(* Logix 5000 Rung export; software revision 33.00 *)

TYPE Banner_IOL_Device :
STRUCT
   Initial_Global_Read : BOOL;
   Command : SINT;
   Data : Banner_IOL_Device_Index;
   Reset : BOOL;
END_STRUCT
END_TYPE

TYPE Banner_IOL_Device_Index :
STRUCT
   Index : Banner_IOL_Device_SubIndex[32];
END_STRUCT
END_TYPE

TYPE Banner_IOL_Device_SubIndex :
STRUCT
   Sub : DINT[34];
END_STRUCT
END_TYPE

TYPE Banner_IOL_Rules :
STRUCT
   Byte_Pos : SINT;   // Byte Position to read from or write data to.
   Multi : SINT;   // Determines if a multiple byte length index is being accessed. Use 2 for 2 bytes length, 3 for 3 byte length, etc..
   Sub_Index : SINT;
   Signed : SINT;   // 0=Unsigned, 1=Signed
END_STRUCT
END_TYPE

TYPE Banner_IOL_Rules_Array :
STRUCT
   Length : DINT;
   Settings : Banner_IOL_Rules_SettingsArray[32];
END_STRUCT
END_TYPE

TYPE Banner_IOL_Rules_SettingsArray :
STRUCT
   Index : DINT;
   Num_Op : INT;   // Number of Operations to read/write Index.
   Total_Bytes : INT;
   RW : SINT;   // 0 = Read Only, 1 = Write Only, 2 = Read or Write
   Rules : Banner_IOL_Rules[34];   // Sub Index Position in IODD.
END_STRUCT
END_TYPE

VAR_GLOBAL   (* controller tags *)
   S100_IOLM1_01 : Banner_IOL_Device;
        .DATA.INDEX[2]   // Direct Parameters 1 (ro)
        .DATA.INDEX[2].SUB[1]   // Reserved
        .DATA.INDEX[2].SUB[2]   // Master Cycle Time
        .DATA.INDEX[2].SUB[3]   // Min Cycle Time
        .DATA.INDEX[2].SUB[4]   // M Sequence Capability
        .DATA.INDEX[2].SUB[5]   // IO-Link Verson ID
        .DATA.INDEX[2].SUB[6]   // Process Data Input Length
        .DATA.INDEX[2].SUB[7]   // Process Data Output Length
        .DATA.INDEX[2].SUB[8]   // Vendor ID
        .DATA.INDEX[2].SUB[9]   // Device ID
        .DATA.INDEX[3]   // Standard Command (wo)
        .DATA.INDEX[3].SUB[1]   // Standard Command
        .DATA.INDEX[4]   // Device Locks
        .DATA.INDEX[4].SUB[1]   // Parameter Access Lock / Data Storage Lock / Local Parameterization Lock / Local User Interface Lock
        .DATA.INDEX[5]   // Serial Number (ro)
        .DATA.INDEX[5].SUB[1]   // SN1
        .DATA.INDEX[5].SUB[2]   // SN2
        .DATA.INDEX[5].SUB[3]   // SN3
        .DATA.INDEX[5].SUB[4]   // SN4
        .DATA.INDEX[5].SUB[5]   // SN5
        .DATA.INDEX[5].SUB[6]   // SN6
        .DATA.INDEX[5].SUB[7]   // SN7
        .DATA.INDEX[5].SUB[8]   // SN8
        .DATA.INDEX[5].SUB[9]   // SN9
        .DATA.INDEX[5].SUB[10]   // SN10
        .DATA.INDEX[5].SUB[11]   // SN11
        .DATA.INDEX[5].SUB[12]   // SN12
        .DATA.INDEX[5].SUB[13]   // SN13
        .DATA.INDEX[5].SUB[14]   // SN14
        .DATA.INDEX[5].SUB[15]   // SN15
        .DATA.INDEX[5].SUB[16]   // SN16
        .DATA.INDEX[6]   // Operating Mode
        .DATA.INDEX[6].SUB[1]   // Operating Mode: 0=Run, 1=4 State Full Logic, 2=Measure, 3=Timer, 4=Counter
        .DATA.INDEX[7]   // Additional Settings
        .DATA.INDEX[7].SUB[1]   // Custom Intensity: 0 to 100%
        .DATA.INDEX[7].SUB[2]   // Custom Flash Rate: 5 to 200 (.5 to 20 Hz)
        .DATA.INDEX[7].SUB[3]   // Custom Display Intensity: 0 to 100 %
        .DATA.INDEX[7].SUB[4]   // Custom Display Scroll Speed: 0 to 255
        .DATA.INDEX[8]   // Display Settings
        .DATA.INDEX[8].SUB[1]   // Text Color / Intensity / Scroll Direction / Scroll Speed / Font Size: see iodd file for more information
        .DATA.INDEX[8].SUB[2]   // Scroll Mode Line 1 / Line 2 / Scynch Scroll / Orientation / Deadspace: see iodd file for more information
        .DATA.INDEX[8].SUB[3]   // Deadspace Value: 0 to 29. The amount of deadspace in columns to insert between the start and end of display strings
        .DATA.INDEX[8].SUB[4]   // Horizontal Justification / Vertial Justification: see iodd file for more information
        .DATA.INDEX[9]   // Timer Settings
        .DATA.INDEX[9].SUB[1]   // Value: Value to count up to or down from.
        .DATA.INDEX[9].SUB[2]   // Timer Unit Type: 0=Days, 1=Hours, 2=Minutes, 3=Seconds, 4=Deci Seconds, 5=Centi Seconds, 6=Milli Seconds
        .DATA.INDEX[9].SUB[3]   // Timer Count Type: 0=Down, 1=Up
        .DATA.INDEX[9].SUB[4]   // Reset Button: 0=Disabled, 1=Button 1, 2=Button 2, 3=Button 3. 4=Button 4, 5=Button 5
        .DATA.INDEX[9].SUB[5]   // Count Inrement Button: 0=Disabled, 1=Button 1, 2=Button 2, 3=Button 3. 4=Button 4, 5=Button 5
        .DATA.INDEX[9].SUB[6]   // Count Decrement Button: 0=Disabled, 1=Button 1, 2=Button 2, 3=Button 3. 4=Button 4, 5=Button 5
        .DATA.INDEX[9].SUB[7]   // Run/Pause Button: 0=Disabled, 1=Button 1, 2=Button 2, 3=Button 3. 4=Button 4, 5=Button 5
        .DATA.INDEX[9].SUB[8]   // Enable Auto Reload: 0=Disabled, 1=Enabled
        .DATA.INDEX[10]   // Measure General Configuration
        .DATA.INDEX[10].SUB[1]   // Filtering: 0=Off, 1=Low, 2=Medium, 3=High
        .DATA.INDEX[10].SUB[2]   // Hysteresis: 0=Off, 1=Low, 2=Medium, 3=High
        .DATA.INDEX[10].SUB[3]   // MTC Mode Data Label 1: DINT representation of a ASCII String
        .DATA.INDEX[10].SUB[4]   // MTC Mode Data Label 2: DINT representation of a ASCII String
        .DATA.INDEX[10].SUB[5]   // MTC Mode Data Label 3: DINT representation of a ASCII String
        .DATA.INDEX[10].SUB[6]   // MTC Mode Data Label 4: DINT representation of a ASCII String
        .DATA.INDEX[10].SUB[7]   // Display Value: 0=Disabled, 1=Enabled
        .DATA.INDEX[10].SUB[8]   // Display Data Label: 0=Disabled, 1=Enabled
        .DATA.INDEX[10].SUB[9]   // Display Bar Graph: 0=Disabled, 1=Enabled
        .DATA.INDEX[10].SUB[10]   // Gauge Mode: 0=Disabled, 1=Enabled
        .DATA.INDEX[10].SUB[11]   // Guage Mode Direction: 0=False, 1=Enabled
        .DATA.INDEX[10].SUB[12]   // Gauge Mode Shift: 0=LED1, 1=LED2, 2=LED3, 3=LED4, 4=LED5, 5=LED6, 6=LED7, 7=LED8, 8=LED9, 9=LED10, 10=LED11, 11=LED12, 12=LED13, 13=LED14, 14=LED15, 15=LED16
        .DATA.INDEX[10].SUB[13]   // Gauge Mode Background Color: 0=Green, 1=Red, 2=Orange, 3=Amber, 4=Yellow, 5=Lime Green, 6=Spring Green, 7=Cyan, 8=Sky Blue, 9=Blue, 10=Violet, 11=Magneta, 12=Rose, 13=White, 14=Custom 1, 15=Cusotm 2
        .DATA.INDEX[10].SUB[14]   // Gauge Mode Background Intensity: 0=High, 1=Medium, 2=Low, 3=Off, 4=Custom
        .DATA.INDEX[10].SUB[15]   // Output Scale Value Low: The lowest number to be displayed
        .DATA.INDEX[10].SUB[16]   // Output Scale Value High: The highest number to be displayed
        .DATA.INDEX[10].SUB[17]   // Input Scale Value Low: The lowest number being input by level mode process data. Set to 0 in timer/counter mode
        .DATA.INDEX[10].SUB[18]   // Input Scale Value High: The highest number being input by level mode porcess data. Set to 65535 in timer/counter mode
        .DATA.INDEX[10].SUB[19]   // Value Label: 4 characters: DINT representation of a ASCII String
        .DATA.INDEX[10].SUB[20]   // Swap Data Label and Value: 0=Disabled, 1=Enabled
        .DATA.INDEX[10].SUB[21]   // MTC Mode Display Orientation: 0=0, 1=180
        .DATA.INDEX[10].SUB[22]   // Bar Graph Height: 1 to 16=Bar Graph Packages
        .DATA.INDEX[10].SUB[23]   // MTC Mode Decimal Places: 0 to 3=Decimal Places
        .DATA.INDEX[10].SUB[24]   // MTC Mode Display as Time: 0=Disabled, 1=Enabled
        .DATA.INDEX[11]   // Measure Base Configuration
        .DATA.INDEX[11].SUB[1]   // Display Override: 0=Disabled, 1=Enabled
        .DATA.INDEX[11].SUB[2]   // Override String Line 1 - 1: Characters 1 to 4. DINT Representation of an ASCII String.
        .DATA.INDEX[11].SUB[3]   // Override String Line 1 - 2: Characters 5 to 8. DINT Representation of an ASCII String.
        .DATA.INDEX[11].SUB[4]   // Override String Line 1 - 3: Characters 9 to 12. DINT Representation of an ASCII String.
        .DATA.INDEX[11].SUB[5]   // Override String Line 1 - 4: Charcter 13. DINT Representation of an ASCII String.
        .DATA.INDEX[11].SUB[6]   // Override String Line 2 - 1: Characters 1 to 4. DINT Representation of an ASCII String.
        .DATA.INDEX[11].SUB[7]   // Override String Line 2 - 2: Characters 5 to 8. DINT Representation of an ASCII String.
        .DATA.INDEX[11].SUB[8]   // Override String Line 2 - 3: Characters 9 to 12. DINT Representation of an ASCII String.
        .DATA.INDEX[11].SUB[9]   // Override String Line 2 - 4: Charcter 13. DINT Representation of an ASCII String.
        .DATA.INDEX[11].SUB[10]   // Animation / Speed / Pulse Pattern: see iodd file for more information
        .DATA.INDEX[11].SUB[11]   // Static Sequence Value: 0 to 255
        .DATA.INDEX[11].SUB[12]   // Sequence Start Location / Top Chevron / Right Chevron / Bottom Chevron / Left Chevron: see iodd file for more information
        .DATA.INDEX[11].SUB[13]   // Color 1 / Color 1 Intensity: see iodd file for more information
        .DATA.INDEX[11].SUB[14]   // Color 2 / Color 2 Intensity: see iodd file for more information
        .DATA.INDEX[11].SUB[15]   // Direction / Haptic Feedback / Audible Type: see iodd file for more information
        .DATA.INDEX[12]   // Measure Threshold 1 Configuration
        .DATA.INDEX[12].SUB[1]   // Threshold Enable: 0=Disabled, 1=Enabled
        .DATA.INDEX[12].SUB[2]   // Threshold Value: 0 to 100 %
        .DATA.INDEX[12].SUB[3]   // Threshold Comparison: 0=Less Than, 1=Greater Than
        .DATA.INDEX[12].SUB[4]   // Threshold Override: 0=Disabled , 1=Enabled
        .DATA.INDEX[12].SUB[5]   // Display Override: 0=Disabled, 1=Enabled
        .DATA.INDEX[12].SUB[6]   // Override String Line 1-1: Characters 1 to 4. DINT representation of an ASCII String.
        .DATA.INDEX[12].SUB[7]   // Override String Line 1-2: Characters 5 to 8. DINT representation of an ASCII String.
        .DATA.INDEX[12].SUB[8]   // Override String Line 1-3: Characters 9 to 12. DINT representation of an ASCII String.
        .DATA.INDEX[12].SUB[9]   // Override String Line 1-4: Character 13. DINT representation of an ASCII String.
        .DATA.INDEX[12].SUB[10]   // Override String Line 2-1: Characters 1 to 4. DINT representation of an ASCII String.
        .DATA.INDEX[12].SUB[11]   // Override String Line 2-2: Characters 5 to 8. DINT representation of an ASCII String.
        .DATA.INDEX[12].SUB[12]   // Override String Line 2-3: Characters 9 to 12. DINT representation of an ASCII String.
        .DATA.INDEX[12].SUB[13]   // Override String Line 2-4: Character 13. DINT representation of an ASCII String.
        .DATA.INDEX[12].SUB[14]   // Animation / Speed / Pulse Pattern: see iodd file for more information
        .DATA.INDEX[12].SUB[15]   // Static Sequence Value: 0 to 255
        .DATA.INDEX[12].SUB[16]   // Sequence Start Location / Top Chevron / Right Chevron / Bottom Chevron / Left Chevron: see iodd file for more information
        .DATA.INDEX[12].SUB[17]   // Color 1 / Color 1 Intensity: see iodd file for more information
        .DATA.INDEX[12].SUB[18]   // Color 2 / Color 2 Intensity: see iodd file for more information
        .DATA.INDEX[12].SUB[19]   // Direction / Haptic Feedback / Audible Type: see iodd fiel for more information
        .DATA.INDEX[13]   // Measure Threshold 2 Configuration
        .DATA.INDEX[13].SUB[1]   // Threshold Enable: 0=Disabled, 1=Enabled
        .DATA.INDEX[13].SUB[2]   // Threshold Value: 0 to 100 %
        .DATA.INDEX[13].SUB[3]   // Threshold Comparison: 0=Less Than, 1=Greater Than
        .DATA.INDEX[13].SUB[4]   // Threshold Override: 0=Disabled , 1=Enabled
        .DATA.INDEX[13].SUB[5]   // Display Override: 0=Disabled, 1=Enabled
        .DATA.INDEX[13].SUB[6]   // Override String Line 1-1: Characters 1 to 4. DINT representation of an ASCII String.
        .DATA.INDEX[13].SUB[7]   // Override String Line 1-2: Characters 5 to 8. DINT representation of an ASCII String.
        .DATA.INDEX[13].SUB[8]   // Override String Line 1-3: Characters 9 to 12 DINT representation of an ASCII String.
        .DATA.INDEX[13].SUB[9]   // Override String Line 1-4: Character 13. DINT representation of an ASCII String.
        .DATA.INDEX[13].SUB[10]   // Override String Line 2-1: Characters 1 to 4. DINT representation of an ASCII String.
        .DATA.INDEX[13].SUB[11]   // Override String Line 2-2: Characters 5 to 8. DINT representation of an ASCII String.
        .DATA.INDEX[13].SUB[12]   // Override String Line 2-3: Characters 9 to 12. DINT representation of an ASCII String.
        .DATA.INDEX[13].SUB[13]   // Override String Line 2-4: Character 13. DINT representation of an ASCII String.
        .DATA.INDEX[13].SUB[14]   // Animation / Speed / Pulse Pattern: see iodd file for more information
        .DATA.INDEX[13].SUB[15]   // Static Sequence Value: 0 to 255
        .DATA.INDEX[13].SUB[16]   // Sequence Start Location / Top Chevron / Right Chevron / Bottom Chevron / Left Chevron: see iodd file for more information
        .DATA.INDEX[13].SUB[17]   // Color 1 / Color 1 Intensity: see iodd file for more information
        .DATA.INDEX[13].SUB[18]   // Color 2 / Color 2 Intensity: see iodd file for more information
        .DATA.INDEX[13].SUB[19]   // Direction / Haptic Feedback / Audible Type: see iodd fiel for more information
        .DATA.INDEX[14]   // Measure Threshold 3 Configuration
        .DATA.INDEX[14].SUB[1]   // Threshold Enable: 0=Disabled, 1=Enabled
        .DATA.INDEX[14].SUB[2]   // Threshold Value: 0 to 100 %
        .DATA.INDEX[14].SUB[3]   // Threshold Comparison: 0=Less Than, 1=Greater Than
        .DATA.INDEX[14].SUB[4]   // Threshold Override: 0=Disabled , 1=Enabled
        .DATA.INDEX[14].SUB[5]   // Display Override: 0=Disabled, 1=Enabled
        .DATA.INDEX[14].SUB[6]   // Override String Line 1-1: Characters 1 to 4. DINT representation of an ASCII String.
        .DATA.INDEX[14].SUB[7]   // Override String Line 1-2: Characters 5 to 8. DINT representation of an ASCII String.
        .DATA.INDEX[14].SUB[8]   // Override String Line 1-3: Characters 9 to 12. DINT representation of an ASCII String.
        .DATA.INDEX[14].SUB[9]   // Override String Line 1-4: Character 13. DINT representation of an ASCII String.
        .DATA.INDEX[14].SUB[10]   // Override String Line 2-1: Characters 1 to 4. DINT representation of an ASCII String.
        .DATA.INDEX[14].SUB[11]   // Override String Line 2-2: Characters 5 to 8. DINT representation of an ASCII String.
        .DATA.INDEX[14].SUB[12]   // Override String Line 2-3: Characters 9 to 12. DINT representation of an ASCII String.
        .DATA.INDEX[14].SUB[13]   // Override String Line 2-4: Character 13. DINT representation of an ASCII String.
        .DATA.INDEX[14].SUB[14]   // Animation / Speed / Pulse Pattern: see iodd file for more information
        .DATA.INDEX[14].SUB[15]   // Static Sequence Value: 0 to 255
        .DATA.INDEX[14].SUB[16]   // Sequence Start Location / Top Chevron / Right Chevron / Bottom Chevron / Left Chevron: see iodd file for more information
        .DATA.INDEX[14].SUB[17]   // Color 1 / Color 1 Intensity: see iodd file for more information
        .DATA.INDEX[14].SUB[18]   // Color 2 / Color 2 Intensity: see iodd file for more information
        .DATA.INDEX[14].SUB[19]   // Direction / Haptic Feedback / Audible Type: see iodd fiel for more information
        .DATA.INDEX[15]   // Measure Threshold 4 Configuration
        .DATA.INDEX[15].SUB[1]   // Threshold Enable: 0=Disabled, 1=Enabled
        .DATA.INDEX[15].SUB[2]   // Threshold Value: 0 to 100 %
        .DATA.INDEX[15].SUB[3]   // Threshold Comparison: 0=Less Than, 1=Greater Than
        .DATA.INDEX[15].SUB[4]   // Threshold Override: 0=Disabled , 1=Enabled
        .DATA.INDEX[15].SUB[5]   // Display Override: 0=Disabled, 1=Enabled
        .DATA.INDEX[15].SUB[6]   // Override String Line 1-1: Characters 1 to 4. DINT representation of an ASCII String.
        .DATA.INDEX[15].SUB[7]   // Override String Line 1-2: Characters 5 to 8. DINT representation of an ASCII String.
        .DATA.INDEX[15].SUB[8]   // Override String Line 1-3: Characters 9 to 12. DINT representation of an ASCII String.
        .DATA.INDEX[15].SUB[9]   // Override String Line 1-4: Character 13. DINT representation of an ASCII String.
        .DATA.INDEX[15].SUB[10]   // Override String Line 2-1: Characters 1 to 4. DINT representation of an ASCII String.
        .DATA.INDEX[15].SUB[11]   // Override String Line 2-2: Characters 5 to 8. DINT representation of an ASCII String.
        .DATA.INDEX[15].SUB[12]   // Override String Line 2-3: Characters 9 to 12. DINT representation of an ASCII String.
        .DATA.INDEX[15].SUB[13]   // Override String Line 2-4: Character 13. DINT representation of an ASCII String.
        .DATA.INDEX[15].SUB[14]   // Animation / Speed / Pulse Pattern: see iodd file for more information
        .DATA.INDEX[15].SUB[15]   // Static Sequence Value: 0 to 255
        .DATA.INDEX[15].SUB[16]   // Sequence Start Location / Top Chevron / Right Chevron / Bottom Chevron / Left Chevron: see iodd file for more information
        .DATA.INDEX[15].SUB[17]   // Color 1 / Color 1 Intensity: see iodd file for more information
        .DATA.INDEX[15].SUB[18]   // Color 2 / Color 2 Intensity: see iodd file for more information
        .DATA.INDEX[15].SUB[19]   // Direction / Haptic Feedback / Audible Type: see iodd fiel for more information
        .DATA.INDEX[16]   // State Parameters 1
        .DATA.INDEX[16].SUB[1]   // Animation / Speed / Pulse Pattern
        .DATA.INDEX[16].SUB[2]   // Static Sequence
        .DATA.INDEX[16].SUB[3]   // Sequence Start Location / Top Chevron / Right Chevron / Bottom Chevron / Left Chevron
        .DATA.INDEX[16].SUB[4]   // Color 1 / Color 1 Intensity
        .DATA.INDEX[16].SUB[5]   // Color 2 / Color 2 Intensity
        .DATA.INDEX[16].SUB[6]   // Direction / Haptic Feedback / Audible Type
        .DATA.INDEX[16].SUB[7]   // Line 1 Text 1: Characters 1 to 4. DINT representation of an ASCII String.
        .DATA.INDEX[16].SUB[8]   // Line 1 Text 2: Characters 5 to 8. DINT representation of an ASCII String.
        .DATA.INDEX[16].SUB[9]   // Line 1 Text 3: Characters 9 to 12. DINT representation of an ASCII String.
        .DATA.INDEX[16].SUB[10]   // Line 1 Text 4: Character 13. DINT representation of an ASCII String.
        .DATA.INDEX[16].SUB[11]   // Line 2 Text 1: Characters 1 to 4. DINT representation of an ASCII String.
        .DATA.INDEX[16].SUB[12]   // Line 2 Text 2: Characters 5 to 8. DINT representation of an ASCII String.
        .DATA.INDEX[16].SUB[13]   // Line 2 Text 3: Characters 9 to 12. DINT representation of an ASCII String.
        .DATA.INDEX[16].SUB[14]   // Line 2 Text 4: Character 13. DINT representation of an ASCII String.
        .DATA.INDEX[17]   // State Parameters 2
        .DATA.INDEX[17].SUB[1]   // Animation / Speed / Pulse Pattern
        .DATA.INDEX[17].SUB[2]   // Static Sequence
        .DATA.INDEX[17].SUB[3]   // Sequence Start Location / Top Chevron / Right Chevron / Bottom Chevron / Left Chevron
        .DATA.INDEX[17].SUB[4]   // Color 1 / Color 1 Intensity
        .DATA.INDEX[17].SUB[5]   // Color 2 / Color 2 Intensity
        .DATA.INDEX[17].SUB[6]   // Direction / Haptic Feedback / Audible Type
        .DATA.INDEX[17].SUB[7]   // Line 1 Text 1: Characters 1 to 4. DINT representation of an ASCII String.
        .DATA.INDEX[17].SUB[8]   // Line 1 Text 2: Characters 5 to 8. DINT representation of an ASCII String.
        .DATA.INDEX[17].SUB[9]   // Line 1 Text 3: Characters 9 to 12. DINT representation of an ASCII String.
        .DATA.INDEX[17].SUB[10]   // Line 1 Text 4: Character 13. DINT representation of an ASCII String.
        .DATA.INDEX[17].SUB[11]   // Line 2 Text 1: Characters 1 to 4. DINT representation of an ASCII String.
        .DATA.INDEX[17].SUB[12]   // Line 2 Text 2: Characters 5 to 8. DINT representation of an ASCII String.
        .DATA.INDEX[17].SUB[13]   // Line 2 Text 3: Characters 9 to 12. DINT representation of an ASCII String.
        .DATA.INDEX[17].SUB[14]   // Line 2 Text 4: Character 13. DINT representation of an ASCII String.
        .DATA.INDEX[18]   // State Parameters 3
        .DATA.INDEX[18].SUB[1]   // Animation / Speed / Pulse Pattern
        .DATA.INDEX[18].SUB[2]   // Static Sequence
        .DATA.INDEX[18].SUB[3]   // Sequence Start Location / Top Chevron / Right Chevron / Bottom Chevron / Left Chevron
        .DATA.INDEX[18].SUB[4]   // Color 1 / Color 1 Intensity
        .DATA.INDEX[18].SUB[5]   // Color 2 / Color 2 Intensity
        .DATA.INDEX[18].SUB[6]   // Direction / Haptic Feedback / Audible Type
        .DATA.INDEX[18].SUB[7]   // Line 1 Text 1: Characters 1 to 4. DINT representation of an ASCII String.
        .DATA.INDEX[18].SUB[8]   // Line 1 Text 2: Characters 5 to 8. DINT representation of an ASCII String.
        .DATA.INDEX[18].SUB[9]   // Line 1 Text 3: Characters 9 to 12. DINT representation of an ASCII String.
        .DATA.INDEX[18].SUB[10]   // Line 1 Text 4: Character 13. DINT representation of an ASCII String.
        .DATA.INDEX[18].SUB[11]   // Line 2 Text 1: Characters 1 to 4. DINT representation of an ASCII String.
        .DATA.INDEX[18].SUB[12]   // Line 2 Text 2: Characters 5 to 8. DINT representation of an ASCII String.
        .DATA.INDEX[18].SUB[13]   // Line 2 Text 3: Characters 9 to 12. DINT representation of an ASCII String.
        .DATA.INDEX[18].SUB[14]   // Line 2 Text 4: Character 13. DINT representation of an ASCII String.
        .DATA.INDEX[19]   // State Parameters 4
        .DATA.INDEX[19].SUB[1]   // Animation / Speed / Pulse Pattern
        .DATA.INDEX[19].SUB[2]   // Static Sequence
        .DATA.INDEX[19].SUB[3]   // Sequence Start Location / Top Chevron / Right Chevron / Bottom Chevron / Left Chevron
        .DATA.INDEX[19].SUB[4]   // Color 1 / Color 1 Intensity
        .DATA.INDEX[19].SUB[5]   // Color 2 / Color 2 Intensity
        .DATA.INDEX[19].SUB[6]   // Direction / Haptic Feedback / Audible Type
        .DATA.INDEX[19].SUB[7]   // Line 1 Text 1: Characters 1 to 4. DINT representation of an ASCII String.
        .DATA.INDEX[19].SUB[8]   // Line 1 Text 2: Characters 5 to 8. DINT representation of an ASCII String.
        .DATA.INDEX[19].SUB[9]   // Line 1 Text 3: Characters 9 to 12. DINT representation of an ASCII String.
        .DATA.INDEX[19].SUB[10]   // Line 1 Text 4: Character 13. DINT representation of an ASCII String.
        .DATA.INDEX[19].SUB[11]   // Line 2 Text 1: Characters 1 to 4. DINT representation of an ASCII String.
        .DATA.INDEX[19].SUB[12]   // Line 2 Text 2: Characters 5 to 8. DINT representation of an ASCII String.
        .DATA.INDEX[19].SUB[13]   // Line 2 Text 3: Characters 9 to 12. DINT representation of an ASCII String.
        .DATA.INDEX[19].SUB[14]   // Line 2 Text 4: Character 13. DINT representation of an ASCII String.
        .DATA.INDEX[20]   // Custom Color 1
        .DATA.INDEX[20].SUB[1]   // Red: 0 to 255
        .DATA.INDEX[20].SUB[2]   // Green: 0 to 255
        .DATA.INDEX[20].SUB[3]   // Blue: 0 to 255
        .DATA.INDEX[21]   // Custom Color 2
        .DATA.INDEX[21].SUB[1]   // Red: 0 to 255
        .DATA.INDEX[21].SUB[2]   // Green: 0 to 255
        .DATA.INDEX[21].SUB[3]   // Blue: 0 to 255
        .DATA.INDEX[22]   // User Input Settings
        .DATA.INDEX[22].SUB[1]   // Touch Sensitivity / Only First Config: see iodd file for more information
        .DATA.INDEX[22].SUB[2]   // Button 1 Function / Mute Enable / Group Override: see iodd file for more information
        .DATA.INDEX[22].SUB[3]   // Button 1 On Delay
        .DATA.INDEX[22].SUB[4]   // Button 2 Function / Mute Enable / Group Override: see iodd file for more information
        .DATA.INDEX[22].SUB[5]   // Button 2 On Delay
        .DATA.INDEX[22].SUB[6]   // Button 3 Function / Mute Enable / Group Override: see iodd file for more information
        .DATA.INDEX[22].SUB[7]   // Button 3 On Delay
        .DATA.INDEX[22].SUB[8]   // Button 4 Function / Mute Enable / Group Override: see iodd file for more information
        .DATA.INDEX[22].SUB[9]   // Button 4 On Delay
        .DATA.INDEX[22].SUB[10]   // Button 5 Function / Mute Enable / Group Override: see iodd file for more information
        .DATA.INDEX[22].SUB[11]   // Button 5 On Delay
        .DATA.INDEX[23]   // Output Settings
        .DATA.INDEX[23].SUB[1]   // Output State: 0=Normally Closed, 1=Normally Open
        .DATA.INDEX[23].SUB[2]   // Button 1 Off Delay Type / Audible Override / Haptic Override: see iodd file for more information
        .DATA.INDEX[23].SUB[3]   // Button 1 Off Delay
        .DATA.INDEX[23].SUB[4]   // Button 2 Off Delay Type / Audible Override / Haptic Override: see iodd file for more information
        .DATA.INDEX[23].SUB[5]   // Button 2 Off Delay
        .DATA.INDEX[23].SUB[6]   // Button 3 Off Delay Type / Audible Override / Haptic Override: see iodd file for more information
        .DATA.INDEX[23].SUB[7]   // Button 3 Off Delay
        .DATA.INDEX[23].SUB[8]   // Button 4 Off Delay Type / Audible Override / Haptic Override: see iodd file for more information
        .DATA.INDEX[23].SUB[9]   // Button 4 Off Delay
        .DATA.INDEX[23].SUB[10]   // Button 5 Off Delay Type / Audible Override / Haptic Override: see iodd file for more information
        .DATA.INDEX[23].SUB[11]   // Button 5 Off Delay
        .DATA.INDEX[24]   // Custom Audible Settings
        .DATA.INDEX[24].SUB[1]   // Custom Type / Custom Sweep Type / Custom Freq 1 / Custom Freq 2: see iodd file for more information
   S100_Rules : Banner_IOL_Rules_Array;
        .SETTINGS[2]   // Direct Parameters 1
        .SETTINGS[2].RULES[0]   // Reserved
        .SETTINGS[2].RULES[1]   // Master Cycle Time
        .SETTINGS[2].RULES[2]   // Min Cycle Time
        .SETTINGS[2].RULES[3]   // M-Sequence Capability
        .SETTINGS[2].RULES[4]   // IO-Link ID
        .SETTINGS[2].RULES[5]   // Process Data Input Length
        .SETTINGS[2].RULES[6]   // Process Data Output Length
        .SETTINGS[2].RULES[7]   // Vendor ID
        .SETTINGS[2].RULES[8]   // Device ID
        .SETTINGS[3]   // Standard Command
        .SETTINGS[3].RULES[0]   // Standard Command
        .SETTINGS[4]   // Device Access Locks
        .SETTINGS[4].RULES[0]   // Parameter Access Locks / Data Storage Lock / Local Parameterization Lock / Local User Interface Lock
        .SETTINGS[5]   // Serial Number
        .SETTINGS[5].RULES[0]   // SN1
        .SETTINGS[5].RULES[1]   // SN2
        .SETTINGS[5].RULES[2]   // SN3
        .SETTINGS[5].RULES[3]   // SN4
        .SETTINGS[5].RULES[4]   // SN5
        .SETTINGS[5].RULES[5]   // SN6
        .SETTINGS[5].RULES[6]   // SN7
        .SETTINGS[5].RULES[7]   // SN8
        .SETTINGS[5].RULES[8]   // SN9
        .SETTINGS[5].RULES[9]   // SN10
        .SETTINGS[5].RULES[10]   // SN11
        .SETTINGS[5].RULES[11]   // SN12
        .SETTINGS[5].RULES[12]   // SN13
        .SETTINGS[5].RULES[13]   // SN14
        .SETTINGS[5].RULES[14]   // SN15
        .SETTINGS[5].RULES[15]   // SN16
        .SETTINGS[6]   // Operating Mode
        .SETTINGS[6].RULES[0]   // Operating Mode
        .SETTINGS[7]   // Additional Settings
        .SETTINGS[7].RULES[0]   // Custom Intensity
        .SETTINGS[7].RULES[1]   // Custom Flash Rate
        .SETTINGS[7].RULES[2]   // Custom Display Intensity
        .SETTINGS[7].RULES[3]   // Custom Display Scroll
        .SETTINGS[8]   // Display Settings
        .SETTINGS[8].RULES[0]   // Text Color / Intensity / Scroll Direction / Scroll Speed
        .SETTINGS[8].RULES[1]   // Scroll Mode Line 1 / Line 2 / Synch Scroll / Orientation / Deadspace
        .SETTINGS[8].RULES[2]   // Deadspace Value
        .SETTINGS[8].RULES[3]   // Horizontal Justificaiton / Vertical Justification
        .SETTINGS[9]   // Timer Counter Settings
        .SETTINGS[9].RULES[0]   // Value
        .SETTINGS[9].RULES[1]   // Timer Unit Type
        .SETTINGS[9].RULES[2]   // Timer Count Type
        .SETTINGS[9].RULES[3]   // Reset Button
        .SETTINGS[9].RULES[4]   // Count Increment Button
        .SETTINGS[9].RULES[5]   // Count Decrement Button
        .SETTINGS[9].RULES[6]   // Run / Pause Button
        .SETTINGS[9].RULES[7]   // Enable Auto Reload
        .SETTINGS[10]   // Measure General Configuration
        .SETTINGS[10].RULES[0]   // Filtering
        .SETTINGS[10].RULES[1]   // Hysteresis
        .SETTINGS[10].RULES[2]   // MTC Mode Data Label 1
        .SETTINGS[10].RULES[3]   // MTC Mode Data Label 2
        .SETTINGS[10].RULES[4]   // MTC Mode Data Label 3
        .SETTINGS[10].RULES[5]   // MTC Mode Data Label 4
        .SETTINGS[10].RULES[6]   // Display Value
        .SETTINGS[10].RULES[7]   // Display Data Label
        .SETTINGS[10].RULES[8]   // Display Bar Graph
        .SETTINGS[10].RULES[9]   // Gauge Mode
        .SETTINGS[10].RULES[10]   // Gauge Mode Direction
        .SETTINGS[10].RULES[11]   // Gauge Mode Shift
        .SETTINGS[10].RULES[12]   // Gauge Mode Background Color
        .SETTINGS[10].RULES[13]   // Gauge Mode Background Intensity
        .SETTINGS[10].RULES[14]   // Output Scale Value Low
        .SETTINGS[10].RULES[15]   // Output Scale Value High
        .SETTINGS[10].RULES[16]   // Input Scale Value Low
        .SETTINGS[10].RULES[17]   // Input Scale Value High
        .SETTINGS[10].RULES[18]   // Value Label
        .SETTINGS[10].RULES[19]   // Swap Data Label and Value
        .SETTINGS[10].RULES[20]   // MTC Mode Display Orientation
        .SETTINGS[10].RULES[21]   // Bar Graph Height
        .SETTINGS[10].RULES[22]   // MTC Mode Decimal Places
        .SETTINGS[10].RULES[23]   // MTC Mode Display as Time
        .SETTINGS[11]   // Measure Base Configuration
        .SETTINGS[11].RULES[0]   // Display Override
        .SETTINGS[11].RULES[1]   // Override String Line 1 - 1
        .SETTINGS[11].RULES[2]   // Override String Line 1 - 2
        .SETTINGS[11].RULES[3]   // Override String Line 1 - 3
        .SETTINGS[11].RULES[4]   // Override String Line 1 - 4
        .SETTINGS[11].RULES[5]   // Override String Line 2 - 1
        .SETTINGS[11].RULES[6]   // Override String Line 2 - 2
        .SETTINGS[11].RULES[7]   // Override String Line 2 - 3
        .SETTINGS[11].RULES[8]   // Override String Line 2 - 4
        .SETTINGS[11].RULES[9]   // Animation / Speed / Pulse Pattern
        .SETTINGS[11].RULES[10]   // Static Sequence Value
        .SETTINGS[11].RULES[11]   // Sequence Start Location / Top Chevron / Right Chevron / Bottom Chevron / Left Chevron
        .SETTINGS[11].RULES[12]   // Color 1 / Color 1 Intensity
        .SETTINGS[11].RULES[13]   // Color 2 / Color 2 Intensity
        .SETTINGS[11].RULES[14]   // Direction / Haptic Feedback / Audible Type
        .SETTINGS[12]   // Measure Threshold 1 Configuration
        .SETTINGS[12].RULES[0]   // Threshold Enable
        .SETTINGS[12].RULES[1]   // Threshold Value
        .SETTINGS[12].RULES[2]   // Threshold Comparison
        .SETTINGS[12].RULES[3]   // Threshold Override
        .SETTINGS[12].RULES[4]   // Display Override
        .SETTINGS[12].RULES[5]   // Override String Line 1 - 1
        .SETTINGS[12].RULES[6]   // Override String Line 1 - 2
        .SETTINGS[12].RULES[7]   // Override String Line 1 - 3
        .SETTINGS[12].RULES[8]   // Override String Line 1 - 4
        .SETTINGS[12].RULES[9]   // Override String Line 2 - 1
        .SETTINGS[12].RULES[10]   // Override String Line 2 - 2
        .SETTINGS[12].RULES[11]   // Override String Line 2 - 3
        .SETTINGS[12].RULES[12]   // Override String Line 2 - 4
        .SETTINGS[12].RULES[13]   // Animation / Speed / Pulse Pattern
        .SETTINGS[12].RULES[14]   // Static Sequence Value
        .SETTINGS[12].RULES[15]   // Sequence Start Location / Top Chevron / Right Chevron / Bottom Chevron / Left Chevron
        .SETTINGS[12].RULES[16]   // Color 1 / Color 1 Intensity
        .SETTINGS[12].RULES[17]   // Color 2 / Color 2 Intensity
        .SETTINGS[12].RULES[18]   // Direction / Haptic Feedback / Audible Type
        .SETTINGS[13]   // Measure Threshold 2 Configuration
        .SETTINGS[13].RULES[0]   // Threshold Enable
        .SETTINGS[13].RULES[1]   // Threshold Value
        .SETTINGS[13].RULES[2]   // Threshold Comparison
        .SETTINGS[13].RULES[3]   // Threshold Override
        .SETTINGS[13].RULES[4]   // Display Override
        .SETTINGS[13].RULES[5]   // Override String Line 1 - 1
        .SETTINGS[13].RULES[6]   // Override String Line 1 - 2
        .SETTINGS[13].RULES[7]   // Override String Line 1 - 3
        .SETTINGS[13].RULES[8]   // Override String Line 1 - 4
        .SETTINGS[13].RULES[9]   // Override String Line 2 - 1
        .SETTINGS[13].RULES[10]   // Override String Line 2 - 2
        .SETTINGS[13].RULES[11]   // Override String Line 2 - 3
        .SETTINGS[13].RULES[12]   // Override String Line 2 - 4
        .SETTINGS[13].RULES[13]   // Animation / Speed / Pulse Pattern
        .SETTINGS[13].RULES[14]   // Static Sequence Value
        .SETTINGS[13].RULES[15]   // Sequence Start Location / Top Chevron / Right Chevron / Bottom Chevron / Left Chevron
        .SETTINGS[13].RULES[16]   // Color 1 / Color 1 Intensity
        .SETTINGS[13].RULES[17]   // Color 2 / Color 2 Intensity
        .SETTINGS[13].RULES[18]   // Direction / Haptic Feedback / Audible Type
        .SETTINGS[14]   // Measure Threshold 3 Configuration
        .SETTINGS[14].RULES[0]   // Threshold Enable
        .SETTINGS[14].RULES[1]   // Threshold Value
        .SETTINGS[14].RULES[2]   // Threshold Comparison
        .SETTINGS[14].RULES[3]   // Threshold Override
        .SETTINGS[14].RULES[4]   // Display Override
        .SETTINGS[14].RULES[5]   // Override String Line 1 - 1
        .SETTINGS[14].RULES[6]   // Override String Line 1 - 2
        .SETTINGS[14].RULES[7]   // Override String Line 1 - 3
        .SETTINGS[14].RULES[8]   // Override String Line 1 - 4
        .SETTINGS[14].RULES[9]   // Override String Line 2 - 1
        .SETTINGS[14].RULES[10]   // Override String Line 2 - 2
        .SETTINGS[14].RULES[11]   // Override String Line 2 - 3
        .SETTINGS[14].RULES[12]   // Override String Line 2 - 4
        .SETTINGS[14].RULES[13]   // Animation / Speed / Pulse Pattern
        .SETTINGS[14].RULES[14]   // Static Sequence Value
        .SETTINGS[14].RULES[15]   // Sequence Start Location / Top Chevron / Right Chevron / Bottom Chevron / Left Chevron
        .SETTINGS[14].RULES[16]   // Color 1 / Color 1 Intensity
        .SETTINGS[14].RULES[17]   // Color 2 / Color 2 Intensity
        .SETTINGS[14].RULES[18]   // Direction / Haptic Feedback / Audible Type
        .SETTINGS[15]   // Measure Threshold 4 Configuration
        .SETTINGS[15].RULES[0]   // Threshold Enable
        .SETTINGS[15].RULES[1]   // Threshold Value
        .SETTINGS[15].RULES[2]   // Threshold Comparison
        .SETTINGS[15].RULES[3]   // Threshold Override
        .SETTINGS[15].RULES[4]   // Display Override
        .SETTINGS[15].RULES[5]   // Override String Line 1 - 1
        .SETTINGS[15].RULES[6]   // Override String Line 1 - 2
        .SETTINGS[15].RULES[7]   // Override String Line 1 - 3
        .SETTINGS[15].RULES[8]   // Override String Line 1 - 4
        .SETTINGS[15].RULES[9]   // Override String Line 2 - 1
        .SETTINGS[15].RULES[10]   // Override String Line 2 - 2
        .SETTINGS[15].RULES[11]   // Override String Line 2 - 3
        .SETTINGS[15].RULES[12]   // Override String Line 2 - 4
        .SETTINGS[15].RULES[13]   // Animation / Speed / Pulse Pattern
        .SETTINGS[15].RULES[14]   // Static Sequence Value
        .SETTINGS[15].RULES[15]   // Sequence Start Location / Top Chevron / Right Chevron / Bottom Chevron / Left Chevron
        .SETTINGS[15].RULES[16]   // Color 1 / Color 1 Intensity
        .SETTINGS[15].RULES[17]   // Color 2 / Color 2 Intensity
        .SETTINGS[15].RULES[18]   // Direction / Haptic Feedback / Audible Type
        .SETTINGS[16]   // State Parameters 1
        .SETTINGS[16].RULES[0]   // Animation / Speed / Pulse Pattern
        .SETTINGS[16].RULES[1]   // Static Sequence Value
        .SETTINGS[16].RULES[2]   // Sequence Start Location / Top Chevron / Right Chevron / Bottom Chevron / Left Chevron
        .SETTINGS[16].RULES[3]   // Color 1 / Color 1 Intensity
        .SETTINGS[16].RULES[4]   // Color 2 / Color 2 Intensity
        .SETTINGS[16].RULES[5]   // Direction / Haptic Feedback / Audible Type
        .SETTINGS[16].RULES[6]   // Line 1 Text 1
        .SETTINGS[16].RULES[7]   // Line 1 Text 2
        .SETTINGS[16].RULES[8]   // Line 1 Text 3
        .SETTINGS[16].RULES[9]   // Line 1 Text 4
        .SETTINGS[16].RULES[10]   // Line 2 Text 1
        .SETTINGS[16].RULES[11]   // Line 2 Text 2
        .SETTINGS[16].RULES[12]   // Line 2 Text 3
        .SETTINGS[16].RULES[13]   // Line 2 Text 4
        .SETTINGS[17]   // State Parameters 2
        .SETTINGS[17].RULES[0]   // Animation / Speed / Pulse Pattern
        .SETTINGS[17].RULES[1]   // Static Sequence Value
        .SETTINGS[17].RULES[2]   // Sequence Start Location / Top Chevron / Right Chevron / Bottom Chevron / Left Chevron
        .SETTINGS[17].RULES[3]   // Color 1 / Color 1 Intensity
        .SETTINGS[17].RULES[4]   // Color 2 / Color 2 Intensity
        .SETTINGS[17].RULES[5]   // Direction / Haptic Feedback / Audible Type
        .SETTINGS[17].RULES[6]   // Line 1 Text 1
        .SETTINGS[17].RULES[7]   // Line 1 Text 2
        .SETTINGS[17].RULES[8]   // Line 1 Text 3
        .SETTINGS[17].RULES[9]   // Line 1 Text 4
        .SETTINGS[17].RULES[10]   // Line 2 Text 1
        .SETTINGS[17].RULES[11]   // Line 2 Text 2
        .SETTINGS[17].RULES[12]   // Line 2 Text 3
        .SETTINGS[17].RULES[13]   // Line 2 Text 4
        .SETTINGS[18]   // State Parameters 3
        .SETTINGS[18].RULES[0]   // Animation / Speed / Pulse Pattern
        .SETTINGS[18].RULES[1]   // Static Sequence Value
        .SETTINGS[18].RULES[2]   // Sequence Start Location / Top Chevron / Right Chevron / Bottom Chevron / Left Chevron
        .SETTINGS[18].RULES[3]   // Color 1 / Color 1 Intensity
        .SETTINGS[18].RULES[4]   // Color 2 / Color 2 Intensity
        .SETTINGS[18].RULES[5]   // Direction / Haptic Feedback / Audible Type
        .SETTINGS[18].RULES[6]   // Line 1 Text 1
        .SETTINGS[18].RULES[7]   // Line 1 Text 2
        .SETTINGS[18].RULES[8]   // Line 1 Text 3
        .SETTINGS[18].RULES[9]   // Line 1 Text 4
        .SETTINGS[18].RULES[10]   // Line 2 Text 1
        .SETTINGS[18].RULES[11]   // Line 2 Text 2
        .SETTINGS[18].RULES[12]   // Line 2 Text 3
        .SETTINGS[18].RULES[13]   // Line 2 Text 4
        .SETTINGS[19]   // State Parameters 4
        .SETTINGS[19].RULES[0]   // Animation / Speed / Pulse Pattern
        .SETTINGS[19].RULES[1]   // Static Sequence Value
        .SETTINGS[19].RULES[2]   // Sequence Start Location / Top Chevron / Right Chevron / Bottom Chevron / Left Chevron
        .SETTINGS[19].RULES[3]   // Color 1 / Color 1 Intensity
        .SETTINGS[19].RULES[4]   // Color 2 / Color 2 Intensity
        .SETTINGS[19].RULES[5]   // Direction / Haptic Feedback / Audible Type
        .SETTINGS[19].RULES[6]   // Line 1 Text 1
        .SETTINGS[19].RULES[7]   // Line 1 Text 2
        .SETTINGS[19].RULES[8]   // Line 1 Text 3
        .SETTINGS[19].RULES[9]   // Line 1 Text 4
        .SETTINGS[19].RULES[10]   // Line 2 Text 1
        .SETTINGS[19].RULES[11]   // Line 2 Text 2
        .SETTINGS[19].RULES[12]   // Line 2 Text 3
        .SETTINGS[19].RULES[13]   // Line 2 Text 4
        .SETTINGS[20]   // Custom Color 1
        .SETTINGS[20].RULES[0]   // Red
        .SETTINGS[20].RULES[1]   // Green
        .SETTINGS[20].RULES[2]   // Blue
        .SETTINGS[21]   // Custom Color 2
        .SETTINGS[21].RULES[0]   // Red
        .SETTINGS[21].RULES[1]   // Green
        .SETTINGS[21].RULES[2]   // Blue
        .SETTINGS[22]   // User Input Settings
        .SETTINGS[22].RULES[0]   // Touch Sensitivity / Only First Config
        .SETTINGS[22].RULES[1]   // Button 1 Function / Mute Enable / Group Override
        .SETTINGS[22].RULES[2]   // Button 1 On Delay
        .SETTINGS[22].RULES[3]   // Button 2 Function / Mute Enable / Group Override
        .SETTINGS[22].RULES[4]   // Button 2 On Delay
        .SETTINGS[22].RULES[5]   // Button 3 Function / Mute Enable / Group Override
        .SETTINGS[22].RULES[6]   // Button 3 On Delay
        .SETTINGS[22].RULES[7]   // Button 4 Function / Mute Enable / Group Override
        .SETTINGS[22].RULES[8]   // Button 4 On Delay
        .SETTINGS[22].RULES[9]   // Button 5 Function / Mute Enable / Group Override
        .SETTINGS[22].RULES[10]   // Button 5 On Delay
        .SETTINGS[23]   // Output Settings
        .SETTINGS[23].RULES[0]   // Output State
        .SETTINGS[23].RULES[1]   // Button 1 Off Delay Type / Audible Override / Haptic Override
        .SETTINGS[23].RULES[2]   // Button 1 Off Delay
        .SETTINGS[23].RULES[3]   // Button 2 Off Delay Type / Audible Override / Haptic Override
        .SETTINGS[23].RULES[4]   // Button 2 Off Delay
        .SETTINGS[23].RULES[5]   // Button 3 Off Delay Type / Audible Override / Haptic Override
        .SETTINGS[23].RULES[6]   // Button 3 Off Delay
        .SETTINGS[23].RULES[7]   // Button 4 Off Delay Type / Audible Override / Haptic Override
        .SETTINGS[23].RULES[8]   // Button 4 Off Delay
        .SETTINGS[23].RULES[9]   // Button 5 Off Delay Type / Audible Override / Haptic Override
        .SETTINGS[23].RULES[10]   // Button 5 Off Delay
        .SETTINGS[24]   // Custom Audible Settings
        .SETTINGS[24].RULES[0]   // Custom Type / Custom Sweep Type / Custom Freq 1 / Custom Freq 2
END_VAR

PROGRAM MainProgram

ROUTINE MainRoutine   (* ladder *)
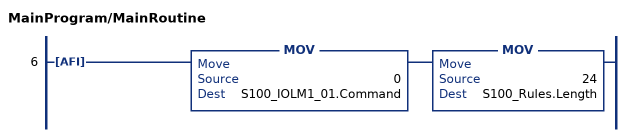
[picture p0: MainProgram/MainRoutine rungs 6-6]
   6: AFI()MOV(0,S100_IOLM1_01.Command)MOV(24,S100_Rules.Length);
END_ROUTINE
END_PROGRAM
